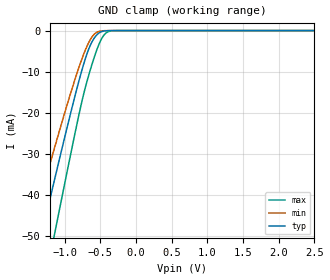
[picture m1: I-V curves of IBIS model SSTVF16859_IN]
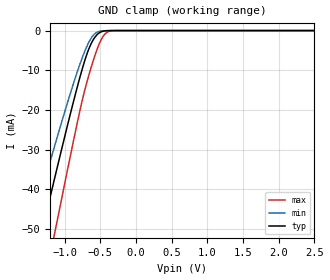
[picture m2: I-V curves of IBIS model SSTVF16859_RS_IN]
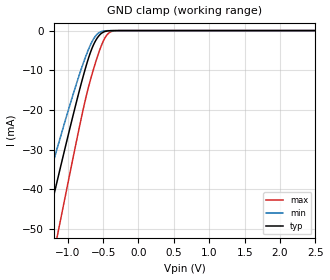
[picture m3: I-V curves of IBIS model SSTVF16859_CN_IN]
| TEXAS INSTRUMENTS INCORPORATED
| Standard Linear and Logic Group
| IBIS Model of SN74SSTVF16859RGQ
| 13-BIT to 26-BIT Registered Buffer w/SSTL2 Input and Outputs
| This file contains package information for the following:
|  QFN 56-pin (RGQ) package as [Component] SSTVF16859_RGQ
| This device can be powered at the following Vccs:
|  2.5 volt Vcc
| This file provides unique models under the [Model Selector] for each Vcc.
| For operation at a specific Vcc, select the appropriate model after each
| [Model Selector] keyword.
[IBIS Ver]   3.2
[Comment char]  |_char
[File Name]   sn74sstvf16859rgq.ibs
[File Rev]   1.1 | X
[Date]   February 10, 2003
[Source]   Data created from TI-SPICE simulations at TI-SLL.
[Notes]   The following is an IBIS list for the SSTVF16859_RGQ.
   Please contact sllibis@ti.com with questions and
   comments concerning SLL IBIS models.
   -As there is no power clamp diode in the Input model,
   we removed the Power Clamp table data from the Input model
   -For differential type input Vinl and Vinh should be
   set as optional, but since IBIS pursers give error, we
   set dummy values of Vinh and Vinl
   -An IBIS model does not adequately simulate the dynamic
   behavior of the multi-stage output driver in the SN74SSTVF16859
   device. TI recommends that customers do NOT use the IBIS model.
   For more accurate simulation results, please use the HSPICE
   model if you can.
[Disclaimer] Property of Texas Instruments Incorporated.  Unauthorized
   reproduction and/or distribution is strictly prohibited.
   This product is protected under copyright law.
   Created  2003, (C) Copyright  2003, Texas Instruments
   Incorporated, All Rights Reserved
   UNLESS THERE IS A SIGNED, WRITTEN AGREEMENT TO THE
   CONTRARY, TEXAS INSTRUMENTS (TI) IS PROVIDING THE IBIS
   MODELS  AND WITHOUT ANY WARRANTY, EXPRESSED OR
   IMPLIED.  TI assumes no liability for:
   1) the accuracy of the IBIS models provided to your
   company;
   2) the proper functioning of these IBIS Models in your
   design or for any resulting applications; or
   3) infringement of patents, copyrights or intellectual
   property rights resulting from your use of these IBIS
   models.
   TI provides IBIS Models as a service to our customers.
   You and your company shall not distribute, sell or give
   these models to anyone else without prior written
   permission from TI.
   TI reserves the right to make changes to our products or
   to discontinue any semiconductor product or service
   without notice, and advises our customers to obtain the
   latest version of relevant information to verify, before
   placing orders, that the information being relied on is
   current.
   Please be aware that your receipt and use of the IBIS
   information provided shall serve as acceptance of these
   terms and conditions.  If you do not accept these terms,
   you should return or destroy the IBIS models and any
   other accompanying information immediately.
| Component SSTVF16859_RGQ 56-pin QFN
[Component]   SSTVF16859_RGQ
[Manufacturer]   Texas Instruments, Inc.
[Package]
|   typ   min   max
R_pkg   7.200e-02   1.900e-02   1.060e-01
L_pkg   2.020e-09   4.150e-10   2.843e-09
C_pkg   3.760e-13   4.000e-14   5.130e-13
[Pin]   signal_name   model_name   R_pin   L_pin   C_pin
50   Q13A   SSTVF16859_OUT   3.700e-02   1.240e-09   2.340e-13
51   Q12A   SSTVF16859_OUT   3.700e-02   1.285e-09   3.260e-13
52   Q11A   SSTVF16859_OUT   4.700e-02   1.462e-09   3.370e-13
53   Q10A   SSTVF16859_OUT   5.900e-02   1.725e-09   3.620e-13
54   Q9A   SSTVF16859_OUT   7.300e-02   2.035e-09   4.000e-13
55   VDDQ   POWER   8.600e-02   2.344e-09   4.550e-13
|   GND   GND   1.020e-01   2.754e-09   4.710e-13
56   Q8A   SSTVF16859_OUT   9.500e-02   2.732e-09   4.790e-13
1   Q7A   SSTVF16859_OUT   9.200e-02   2.609e-09   4.830e-13
2   Q6A   SSTVF16859_OUT   8.900e-02   2.525e-09   4.670e-13
3   Q5A   SSTVF16859_OUT   8.700e-02   2.459e-09   4.370e-13
4   Q4A   SSTVF16859_OUT   8.600e-02   2.423e-09   4.460e-13
5   Q3A   SSTVF16859_OUT   8.500e-02   2.417e-09   4.750e-13
6   Q2A   SSTVF16859_OUT   8.500e-02   2.370e-09   4.140e-13
|   GND   GND   8.500e-02   2.372e-09   4.020e-13
7   Q1A   SSTVF16859_OUT   8.600e-02   2.430e-09   4.660e-13
8   Q13B   SSTVF16859_OUT   8.700e-02   2.448e-09   4.500e-13
9   VDDQ   POWER   8.900e-02   2.494e-09   4.400e-13
10   Q12B   SSTVF16859_OUT   9.100e-02   2.571e-09   4.710e-13
11   Q11B   SSTVF16859_OUT   9.400e-02   2.665e-09   4.880e-13
12   Q10B   SSTVF16859_OUT   9.800e-02   2.796e-09   4.850e-13
13   Q9B   SSTVF16859_OUT   1.060e-01   2.843e-09   4.550e-13
14   Q8B   SSTVF16859_OUT   9.200e-02   2.478e-09   4.610e-13
15   Q7B   SSTVF16859_OUT   7.600e-02   2.102e-09   4.240e-13
16   Q6B   SSTVF16859_OUT   6.300e-02   1.827e-09   3.720e-13
|   GND   GND   5.200e-02   1.568e-09   3.460e-13
17   VDDQ   POWER   4.300e-02   1.405e-09   3.390e-13
18   Q5B   SSTVF16859_OUT   3.800e-02   1.236e-09   2.660e-13
19   Q4B   SSTVF16859_OUT   3.800e-02   1.234e-09   2.610e-13
20   Q3B   SSTVF16859_OUT   4.000e-02   1.336e-09   3.310e-13
21   Q2B   SSTVF16859_OUT   4.700e-02   1.467e-09   3.340e-13
22   Q1B   SSTVF16859_OUT   5.900e-02   1.723e-09   3.580e-13
23   VDDQ   POWER   7.200e-02   2.021e-09   3.900e-13
|   GND   GND   8.600e-02   2.341e-09   4.480e-13
24   D1   SSTVF16859_IN   1.020e-01   2.753e-09   4.650e-13
25   D2   SSTVF16859_IN   9.500e-02   2.732e-09   4.820e-13
26   VCC   POWER   9.200e-02   2.607e-09   5.010e-13
27   VDDQ   POWER   9.100e-02   2.551e-09   4.900e-13
|   GND   GND   8.800e-02   2.476e-09   4.410e-13
28   D3   SSTVF16859_IN   8.700e-02   2.451e-09   4.500e-13
29   D4   SSTVF16859_IN   8.600e-02   2.432e-09   4.720e-13
30   D5   SSTVF16859_IN   8.500e-02   2.372e-09   4.080e-13
|   GND   GND   8.500e-02   2.371e-09   4.080e-13
31   D6   SSTVF16859_IN   8.600e-02   2.429e-09   4.720e-13
32   VREF   SSTVF16859_VR_IN   8.700e-02   2.446e-09   4.560e-13
33   VCC   POWER   8.900e-02   2.493e-09   4.440e-13
34   VDDQ   POWER   9.100e-02   2.560e-09   4.920e-13
35   CLK   SSTVF16859_CP_IN   9.300e-02   2.629e-09   5.130e-13
36   CLK_   SSTVF16859_CN_IN   9.700e-02   2.776e-09   4.910e-13
37   GND   GND   1.060e-01   2.834e-09   4.530e-13
38   RESET_   SSTVF16859_RS_IN   8.600e-02   2.338e-09   4.500e-13
39   D7   SSTVF16859_IN   7.200e-02   2.023e-09   4.050e-13
40   D8   SSTVF16859_IN   5.900e-02   1.715e-09   3.680e-13
|   GND   GND   4.700e-02   1.460e-09   3.400e-13
41   D9   SSTVF16859_IN   4.100e-02   1.356e-09   3.420e-13
42   D10   SSTVF16859_IN   3.700e-02   1.205e-09   2.310e-13
43   D11   SSTVF16859_IN   4.100e-02   8.970e-10   1.050e-13
|   GND   GND   3.700e-02   8.170e-10   8.100e-14
44   VDDQ   POWER   3.700e-02   8.090e-10   9.800e-14
45   VCC   POWER   1.900e-02   4.150e-10   4.000e-14
46   D12   SSTVF16859_IN   4.100e-02   8.960e-10   1.020e-13
47   D13   SSTVF16859_IN   4.000e-02   8.900e-10   9.000e-14
48   GND   GND   4.100e-02   8.990e-10   9.500e-14
49   VDDQ   POWER   4.000e-02   8.870e-10   8.900e-14
| Models and submodels in the file (6): SSTVF16859_IN (Input), SSTVF16859_RS_IN (Input), SSTVF16859_CN_IN (Input), SSTVF16859_CP_IN (Input), SSTVF16859_VR_IN (Input), SSTVF16859_OUT (Output)
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| NOTE:  The [Diff Pin] section is commented out because the ibischk3 program
|   currently flags it as an Error when it shouldn't
| NOTE2: This differential info is for the 64 pin DGG package, NOT for the 56
|   pin QFN package
| [Diff Pin]  inv_pin   vdiff   tdelay_typ
|48   49   0.180   0
|35   45   0.310   0
|36   45   0.310   0
|40   45   0.310   0
|41   45   0.310   0
|42   45   0.310   0
|44   45   0.310   0
|52   45   0.310   0
|53   45   0.310   0
|55   45   0.310   0
|56   45   0.310   0
|57   45   0.310   0
|61   45   0.310   0
|62   45   0.310   0
[Model]   SSTVF16859_IN
Model_type  Input
Vinh=0.97
Vinl=1.53
| variable   typ   min   max
C_comp   2.70pF   2.60pF   2.80pF
[Temperature Range]   40   85   0
| Ambient temperature   25   70   0
[Voltage range]   2.5   2.5   2.5
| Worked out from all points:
|   GND clamp passes 1 mA (typ) near -0.55 V on its own axis
[GND Clamp]
| SSTVF16859_IN
|   Voltage   I(typ)   I(min)   I(max)
-2.5V     -138.9mA   -116.4mA   -166.4mA
-1.49V    -62.29mA   -50.36mA   -79.78mA
-1.44V    -58.54mA   -47.18mA   -75.45mA
-1.305V   -48.45mA   -38.68mA   -63.77mA
-1.14V    -36.26mA   -28.51mA   -49.49mA
-1.1V     -33.34mA   -26.09mA   -46.04mA
-750mV    -9.216mA   -6.589mA   -16.74mA
-655mV    -4.225mA   -2.699mA   -10.49mA
-555mV    -1.172mA   -492.4uA   -5.026mA
-445mV    -108.7uA   -34uA      -1.041mA
-325mV    -3.339uA   -1.231uA   -42.72uA
2.5V      313.9pA    204.1pA    3.455nA
[Model]   SSTVF16859_RS_IN
Model_type  Input
Vinl=0.7
Vinh=1.7
| variable   typ   min   max
C_comp   2.59pF   2.18pF   3.00pF
[Temperature Range]   40   85   0
| Ambient temperature   25   70   0
[Voltage range]   2.5   2.3   2.7
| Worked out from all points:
|   GND clamp passes 1 mA (typ) near -0.54 V on its own axis
[GND Clamp]
| SSTVF16859_RS_IN
|   Voltage   I(typ)   I(min)   I(max)
-2.5V     -142.5mA   -119mA     -171.5mA
-1.49V    -63.97mA   -51.46mA   -82.34mA
-1.44V    -60.12mA   -48.21mA   -77.9mA
-1.305V   -49.78mA   -39.54mA   -65.87mA
-1.14V    -37.28mA   -29.15mA   -51.17mA
-910mV    -20.37mA   -15.32mA   -30.82mA
-745mV    -9.239mA   -6.51mA    -17.05mA
-650mV    -4.192mA   -2.605mA   -10.64mA
-550mV    -1.134mA   -458.4uA   -5.008mA
-445mV    -115.2uA   -35.68uA   -1.098mA
-325mV    -3.541uA   -1.298uA   -45.32uA
2.5V      338.1pA    223.4pA    3.669nA
[Model]   SSTVF16859_CN_IN
Model_type  Input
Vinh=0.97
Vinl=1.53
| variable   typ   min   max
C_comp   2.56pF   2.50pF   2.61pF
[Temperature Range]   40   85   0
| Ambient temperature   25   70   0
[Voltage range]   2.5   2.3   2.7
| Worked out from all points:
|   GND clamp passes 1 mA (typ) near -0.54 V on its own axis
[GND Clamp]
| SSTVF16859_CN_IN
|   Voltage   I(typ)   I(min)   I(max)
-2.5V     -142.5mA   -119mA     -171.5mA
-1.49V    -63.97mA   -51.46mA   -82.34mA
-1.44V    -60.12mA   -48.21mA   -77.9mA
-1.305V   -49.78mA   -39.54mA   -65.87mA
-1.14V    -37.28mA   -29.15mA   -51.17mA
-910mV    -20.37mA   -15.32mA   -30.82mA
-745mV    -9.239mA   -6.51mA    -17.05mA
-650mV    -4.192mA   -2.605mA   -10.64mA
-550mV    -1.134mA   -458.4uA   -5.008mA
-445mV    -115.2uA   -35.68uA   -1.098mA
-325mV    -3.541uA   -1.298uA   -45.32uA
2.5V      338.1pA    223.4pA    3.669nA
